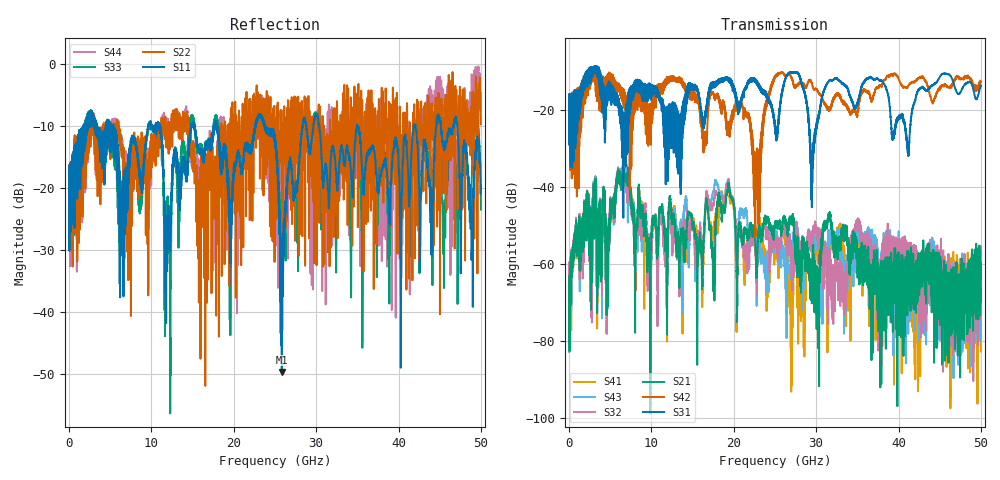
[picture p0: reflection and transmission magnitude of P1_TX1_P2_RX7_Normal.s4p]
!Keysight Technologies,N5225B,MY57041031,A.13.20.10
!Date: Friday, May 31, 2019 11:38:23
!Correction: S11(Full 4 Port(1,2,3,4))
!S12(Full 4 Port(1,2,3,4))
!S13(Full 4 Port(1,2,3,4))
!S14(Full 4 Port(1,2,3,4))
!S21(Full 4 Port(1,2,3,4))
!S22(Full 4 Port(1,2,3,4))
!S23(Full 4 Port(1,2,3,4))
!S24(Full 4 Port(1,2,3,4))
!S31(Full 4 Port(1,2,3,4))
!S32(Full 4 Port(1,2,3,4))
!S33(Full 4 Port(1,2,3,4))
!S34(Full 4 Port(1,2,3,4))
!S41(Full 4 Port(1,2,3,4))
!S42(Full 4 Port(1,2,3,4))
!S43(Full 4 Port(1,2,3,4))
!S44(Full 4 Port(1,2,3,4))
!S4P File: Measurements: <S11,S12,S13,S14>,
!<S21,S22,S23,S24>,
!<S31,S32,S33,S34>,
!<S41,S42,S43,S44>:
# Hz S  dB  R 50.0
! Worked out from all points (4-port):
!   5000 points, 10 MHz to 50 GHz, reference 50 ohm
!   strongest paths, dB at 10 MHz, 12.51 GHz, 25.01 GHz, 37.51 GHz, 50 GHz:
!     S31: -19.4, -29.2, -24.6, -11.8, -13.5
!     S42: -19.4, -12.2, -11.6, -13.9, -12.6
!     S21: -63.1, -47.2, -50.5, -67.5, -63.1
!     S32: -59.5, -51.2, -54.3, -65.1, -67.6
!     S43: -75.9, -50.2, -53.3, -59.3, -72.1
!     S41: -64.6, -47.6, -57.2, -76.3, -82.7
!   lowest |S11| = -49.7 dB at 25.83 GHz (marker M1), VSWR 1.01, Z = 50 + j0.326 ohm
!   |S11| at or under -10 dB: 18.01 GHz to 22.61 GHz (4.597 GHz wide, 22.6 % of centre); 30.38 GHz to 34.94 GHz (4.563 GHz wide, 14 % of centre); 34.97 GHz to 41.82 GHz (6.84 GHz wide, 17.8 % of centre)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
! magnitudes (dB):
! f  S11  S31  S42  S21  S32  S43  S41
! 10 MHz  -19.9  -19.4  -19.4  -63.1  -59.5  -75.9  -64.6
! 6.14 GHz  -20.5  -20.5  -13.8  -36.0  -35.6  -35.2  -35.5
! 9.71 GHz  -9.7  -16.1  -24.7  -55.2  -53.6  -53.0  -54.4
! 22.81 GHz  -8.8  -12.8  -36.0  -60.2  -68.0  -64.7  -52.2
! 25.83 GHz  -49.7  -16.0  -10.2  -51.0  -50.9  -55.7  -50.6
! 28.56 GHz  -8.6  -15.0  -13.4  -57.1  -55.9  -61.2  -64.3
! 50 GHz  -19.7  -13.5  -12.6  -63.1  -67.6  -72.1  -82.7
